INTERFACE ITF_Axis_Ex EXTENDS ITF_Axis

METHOD M_Cyclic : BOOL
VAR_INPUT
END_VAR
END_METHOD

METHOD M_Home : BOOL
VAR_INPUT
	Execute:BOOL;
END_VAR
END_METHOD

METHOD M_Reset : BOOL
VAR_INPUT
	Execute:BOOL;

	
END_VAR
END_METHOD

END_INTERFACE
